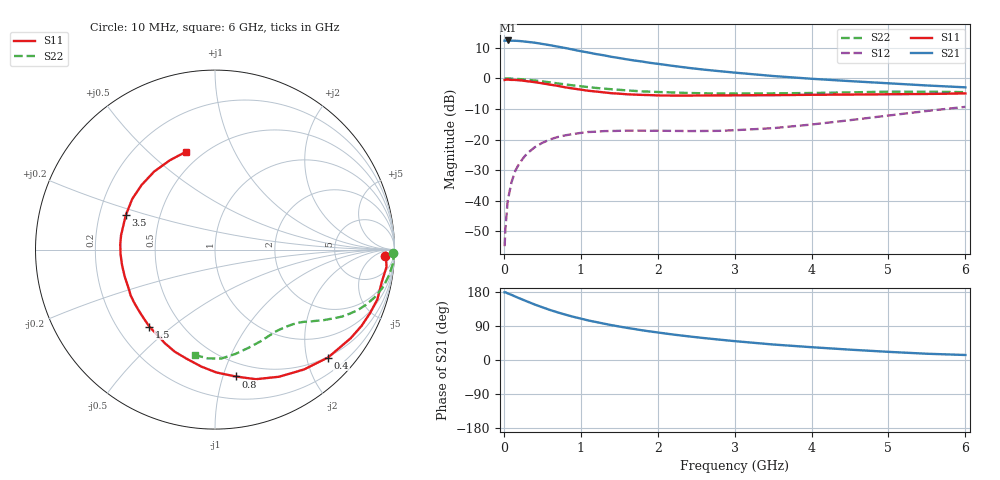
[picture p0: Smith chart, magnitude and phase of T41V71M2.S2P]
! Infineon Technologies  Discrete & RF Semiconductors
! BFR182T
! Si NPN RF Bipolar Junction Transistor in SC75
! VCE = 1.75 V  IC = 1.2 mA
! Common Emitter S-Parameters:  October  1999
# GHz  S  MA  R  50
!  f  S11  S21  S12  S22
! GHz  MAG  ANG  MAG  ANG  MAG  ANG  MAG  ANG
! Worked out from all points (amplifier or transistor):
!   36 points, 10 MHz to 6 GHz, reference 50 ohm
!   highest |S21| = 12.4 dB at 50 MHz (marker M1)
!   |S21| within 3 dB of that: start of sweep to 900.4 MHz
!   unconditionally stable (mu >= 1): 2.26 GHz to 4.563 GHz
!   at 250 MHz: K = 0.10, MSG = 19.1 dB, |S12| = -26.1 dB
!   at 1.4 GHz: K = 0.64, MSG = 12.1 dB, |S12| = -17.2 dB
!   at 6 GHz: K = 0.85, MSG = 3.2 dB, |S12| = -9.3 dB
!   S11 on the Smith chart (normalised r, x): 10 MHz: 24, -17; 400 MHz: 0.48, -2.41; 800 MHz: 0.38, -1.10; 1.5 GHz: 0.33, -0.42; 3.5 GHz: 0.31, +0.17; 6 GHz: 0.41, +0.66
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0.01  0.9455 -2.2  4.153 178.6  0.0018 83.6  0.9914 -1.2
0.02  0.9519 -1.0  4.145 178.8  0.0034 98.2  0.9999 -1.0
0.05  0.9604 -5.8  4.19 175.8  0.01 91.7  0.9959 -2.3
0.1  0.9466 -10.9  4.148 171.9  0.0201 84.0  0.9948 -4.5
0.15  0.9464 -17.1  4.141 167.3  0.0311 80.0  0.9854 -6.7
0.25  0.9205 -27.5  4.051 158.9  0.0494 73.9  0.9669 -11.0
0.4  0.8706 -43.7  3.854 146.5  0.0747 65.2  0.9269 -16.8
0.5  0.8318 -53.4  3.675 139.2  0.0883 60.1  0.8963 -20.0
0.6  0.7935 -63.2  3.502 132.0  0.1005 55.3  0.8637 -23.0
0.7  0.7571 -72.5  3.321 125.7  0.1101 51.4  0.8304 -25.5
0.8  0.716 -80.8  3.149 119.7  0.1174 47.7  0.7996 -27.8
0.9  0.6845 -89.4  2.967 114.2  0.1232 44.2  0.7704 -29.7
1.1  0.6285 -104.5  2.658 104.2  0.1331 39.2  0.7218 -33.0
1.3  0.5918 -118.1  2.395 96.0  0.1375 35.7  0.6819 -35.7
1.5  0.5637 -130.5  2.16 88.4  0.1391 33.5  0.6525 -38.0
1.8  0.5385 -147.0  1.89 78.3  0.1401 31.6  0.6152 -41.6
2.2  0.525 -163.6  1.606 67.2  0.1387 32.2  0.5898 -46.1
2.8  0.5286 176.9  1.318 53.8  0.139 37.6  0.5671 -54.2
3.5  0.5327 159.0  1.097 40.9  0.1537 47.4  0.5708 -63.8
4.5  0.545 138.5  0.905 27.3  0.2077 57.1  0.5923 -78.9
5.5  0.5577 116.8  0.768 16.5  0.2937 57.5  0.6073 -94.0
6  0.5688 106.4  0.716 13.2  0.3433 54.7  0.5974 -101.0
